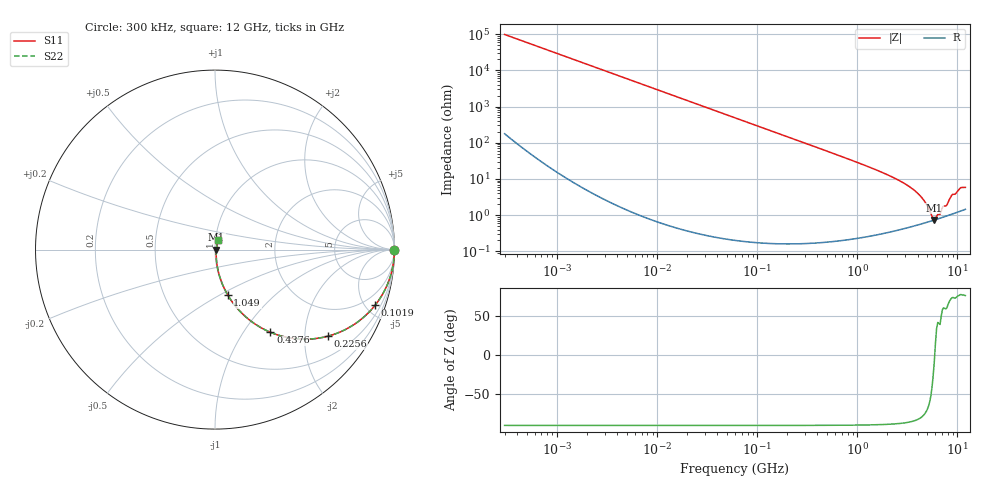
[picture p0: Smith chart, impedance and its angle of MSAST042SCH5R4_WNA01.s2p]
! MSAST042SCH5R4_WNA01  S-PARAMETER MODEL  ( General Type )
! Model Generated by TAIYO YUDEN Corporation (http://www.ty-top.com)
! Version 1.0
! TAIYO YUDEN Control No. 150820
! Copyright(c) 2015 TAIYO YUDEN CO.,LTD. All Rights Reserved.
! Product Description (link to TY-COMPAS)
! https://ds.yuden.co.jp/TYCOMPAS/or/detail?pn=MSAST042SCH5R4BWNA01&u=M
! Products Name : Multilayer Ceramic Capacitors
! Characteristics :
!  Capacitance : 5.4 pF , Rated Voltage : 25V , TCC : CH / C0H
!  Case Size : 0.4 x 0.2 / 0.016 x 0.008 [mm/inch] , Thickness : 0.2 / 0.008 [mm/inch]
!  (Conditions: Temperature = 25 degC , DC Bias Current/Voltage = 0A / 0V)
! External Node Assignments :
!  1  o---| |---o  2
! GND o---------o GND
! Frequency Range : 0.3MHz  -  12000MHz  [ 401 STEP ]
# MHz S RI R 50
! Freq[MHz].  S11 Real  S11 Imag  S21 Real  S21 Imag  S12 Real  S12 Imag  S22 Real  S22 Imag
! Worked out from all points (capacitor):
!   401 points, 300 kHz to 12 GHz, reference 50 ohm
!   read as one part in series: C = 5.41 pF near 316.3 kHz
!   lowest |Z| = 741 mohm at 5.869 GHz (marker M1)
!   series resonance near 5.927 GHz, so ESL is about 130 pH
!   S11 on the Smith chart (normalised r, x): 300 kHz: open; 101.9 MHz: 1.00, -5.77; 225.6 MHz: 1.00, -2.60; 437.6 MHz: 1.00, -1.34; 1.049 GHz: 1.00, -0.54; 12 GHz: 1.03, +0.11
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0.3  1 -0.00102  2.88e-06 0.00102  2.88e-06 0.00102  1 -0.00102
1.769972  1 -0.00602  3.84e-05 0.00602  3.84e-05 0.00602  1 -0.00602
10.44266  0.9987 -0.0355  0.00127 0.0355  0.00127 0.0355  0.9987 -0.0355
27.82928  0.9911 -0.0938  0.00891 0.0938  0.00891 0.0938  0.9911 -0.0938
60  0.9599 -0.1959  0.0401 0.1959  0.0401 0.1959  0.9599 -0.1959
101.9188  0.8925 -0.3094  0.1075 0.3094  0.1075 0.3094  0.8925 -0.3094
151.6462  0.7894 -0.4073  0.2106 0.4073  0.2106 0.4073  0.7894 -0.4073
225.6362  0.6285 -0.4826  0.3715 0.4826  0.3715 0.4826  0.6285 -0.4826
353.9943  0.4067 -0.4902  0.5933 0.4902  0.5933 0.4902  0.4067 -0.4902
437.5599  0.3092 -0.4609  0.6908 0.4609  0.6908 0.4609  0.3092 -0.4609
668.5285  0.1597 -0.3641  0.8403 0.3641  0.8403 0.3641  0.1597 -0.3641
1048.836  0.0705 -0.2518  0.9295 0.2518  0.9295 0.2518  0.0705 -0.2518
2088.533  0.0182 -0.1206  0.9818 0.1206  0.9818 0.1206  0.0182 -0.1206
3026.31  0.00937 -0.0708  0.9906 0.0708  0.9906 0.0708  0.00937 -0.0708
3944.255  0.00694 -0.041  0.9931 0.041  0.9931 0.041  0.00694 -0.041
4623.766  0.00656 -0.0246  0.9934 0.0246  0.9934 0.0246  0.00656 -0.0246
5565.855  0.00698 -0.00617  0.993 0.00617  0.993 0.00617  0.00698 -0.00617
5868.704  0.00727 -0.00111  0.9927 0.00111  0.9927 0.00111  0.00727 -0.00111
6354.153  0.00783 0.00681  0.9922 -0.00681  0.9922 -0.00681  0.00783 0.00681
8732.115  0.0115 0.0324  0.9885 -0.0324  0.9885 -0.0324  0.0115 0.0324
10793.46  0.0158 0.0545  0.9842 -0.0545  0.9842 -0.0545  0.0158 0.0545
12000  0.0173 0.0548  0.9827 -0.0548  0.9827 -0.0548  0.0173 0.0548
